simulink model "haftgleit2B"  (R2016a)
settings: Solver=ode45  SolverMode=SingleTasking  StartTime=0.0  StopTime=4  RelTol=1e-6  AbsTol=1e-6
undefined symbols (not defined in the file or in its folder): FN, mug, muh
libraries: simulink x1

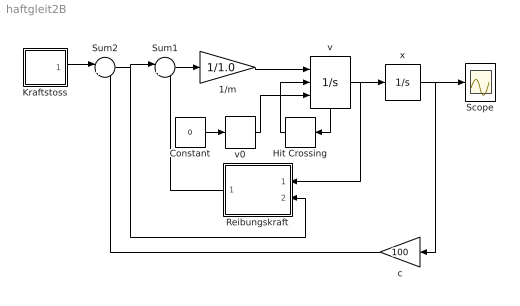
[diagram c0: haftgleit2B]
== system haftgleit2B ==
  note: .
  1/m : Gain  Gain=1/1.0
  Constant : Constant  Value=0
  Hit Crossing : HitCross
  Kraftstoss : Subsystem
  Reibungskraft : Subsystem
  Scope : Scope
  Sum1 : Sum  Inputs=|++
  Sum2 : Sum  Inputs=|+-
  c : Gain  Gain=100
  v : Integrator  ExternalReset=rising  InitialConditionSource=external  ShowStatePort=on
  v0 : InitialCondition  Value=-30
  x : Integrator  InitialCondition=3.5  UpperSaturationLimit=100  LowerSaturationLimit=-100
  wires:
  x/1 -> Scope/1, c/1
  Sum1/1 -> 1/m/1
  v/1 -> Reibungskraft/1(v), x/1
  1/m/1 -> v/1
  Reibungskraft/1(F_R) -> Sum1/2
  c/1 -> Sum2/2
  Kraftstoss/1(Fext) -> Sum2/1
  Sum2/1 -> Sum1/1, Reibungskraft/2(F_ext)
  Hit Crossing/1 -> v/2
  v/State -> Hit Crossing/1
  Constant/1 -> v0/1
  v0/1 -> v/3

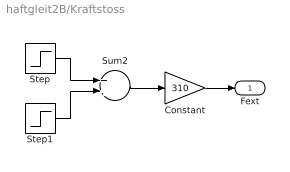
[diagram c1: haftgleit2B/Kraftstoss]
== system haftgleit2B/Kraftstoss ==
  Constant : Gain  Gain=310
  Step : Step  Time=1.5  SampleTime=0
  Step1 : Step  Time=1.6  After=-1  SampleTime=0
  Sum2 : Sum
  Fext : Outport
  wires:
  Constant/1 -> Fext/1
  Step1/1 -> Sum2/2
  Step/1 -> Sum2/1
  Sum2/1 -> Constant/1

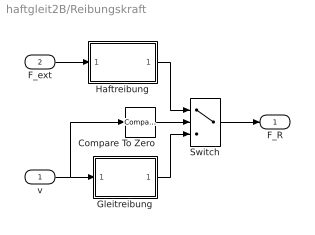
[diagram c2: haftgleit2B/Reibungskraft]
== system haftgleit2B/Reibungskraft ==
  v : Inport
  F_ext : Inport  Port=2
  Compare To Zero : simulink/Logic and Bit Operations/Compare To Zero  SystemSampleTime=-1  relop===  LogicOutDataTypeMode=uint8
  Gleitreibung : Subsystem
  Haftreibung : Subsystem
  Switch : Switch  Criteria=u2 ~= 0  Threshold=0.5
  F_R : Outport
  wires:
  Switch/1 -> F_R/1
  F_ext/1 -> Haftreibung/1(F_ext)
  v/1 -> Compare To Zero/1, Gleitreibung/1(v)
  Haftreibung/1(F_h) -> Switch/1
  Gleitreibung/1(F_g) -> Switch/3
  Compare To Zero/1 -> Switch/2

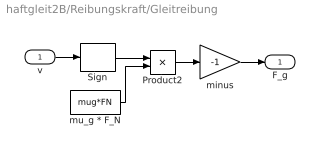
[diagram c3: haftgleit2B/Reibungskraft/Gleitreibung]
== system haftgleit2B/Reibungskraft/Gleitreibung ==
  v : Inport
  Product2 : Product
  Sign : Signum
  minus : Gain  Gain=-1
  mu_g * F_N : Constant  Value=mug*FN
  F_g : Outport
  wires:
  mu_g * F_N/1 -> Product2/2
  Sign/1 -> Product2/1
  v/1 -> Sign/1
  Product2/1 -> minus/1
  minus/1 -> F_g/1

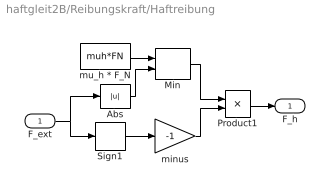
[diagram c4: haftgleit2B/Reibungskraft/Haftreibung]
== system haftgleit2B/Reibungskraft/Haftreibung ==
  F_ext : Inport
  Abs : Abs
  Min : MinMax  Inputs=2
  Product1 : Product
  Sign1 : Signum
  minus : Gain  Gain=-1
  mu_h * F_N : Constant  Value=muh*FN
  F_h : Outport
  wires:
  Abs/1 -> Min/2
  mu_h * F_N/1 -> Min/1
  Min/1 -> Product1/1
  F_ext/1 -> Abs/1, Sign1/1
  Product1/1 -> F_h/1
  Sign1/1 -> minus/1
  minus/1 -> Product1/2
